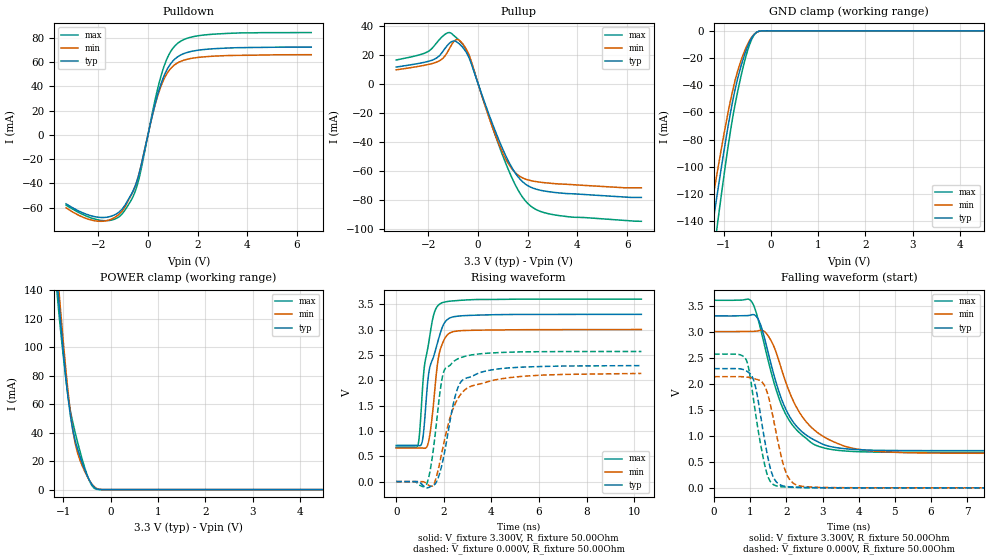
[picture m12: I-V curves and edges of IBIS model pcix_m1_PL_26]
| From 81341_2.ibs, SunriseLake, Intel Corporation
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[Model]   pcix_m1_PL_26
Model_type   I/O
Vinl = 1.155V
Vinh = 1.650V
Vmeas = 1.320V
Vref = 0.000V
Cref = 10.000pF
Rref = 25.000Ohm
|   typ   min   max
C_comp   7.5000pF   6.000pF   9.000pF
[Voltage Range]   3.300V   3.000V   3.600V
[Temperature Range]   60.0   110.0   -5.0
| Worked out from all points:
|   slope of the pulldown table from 0 to 0.495 V, typ, clamps not added: 12.3 ohm
|   slope of the pullup table from 0 to 0.495 V, typ, clamps not added: 20.8 ohm
|   GND clamp passes 1 mA (typ) near -0.30 V on its own axis
|   POWER clamp passes 1 mA (typ) near -0.32 V on its own axis
|   falling waveform, V_fixture 3.300V, R_fixture 50.00Ohm: 20-80 % time 796ps typ, 991ps min, 811ps max; typ from 3.3 V to 0.714 V
|   rising waveform, V_fixture 3.300V, R_fixture 50.00Ohm: 20-80 % time 563ps typ, 338ps min, 429ps max; typ from 0.714 V to 3.3 V
|   rising waveform, V_fixture 0.000V, R_fixture 50.00Ohm: 20-80 % time 596ps typ, 835ps min, 410ps max; typ from 0 V to 2.29 V
|   falling waveform, V_fixture 0.000V, R_fixture 50.00Ohm: 20-80 % time 349ps typ, 405ps min, 362ps max; typ from 2.29 V to 0 V
[Pulldown]
|   Voltage   I(typ)   I(min)   I(max)
-3.3V     -56.89mA   -60.17mA   -57.97mA
-1.9V     -68.16mA   -71.31mA   -70.53mA
-1.35V    -66.03mA   -68.25mA   -69.58mA
-950mV    -58.67mA   -60.17mA   -62.73mA
-600mV    -46.21mA   -46.47mA   -50.78mA
-400mV    -35.07mA   -34.98mA   -39.08mA
200mV     18.27mA    17.98mA    20.69mA
500mV     40.57mA    38.9mA     46.82mA
850mV     56.8mA     53.13mA    66.45mA
1.25V     65.06mA    59.98mA    76.34mA
2.65V     71.02mA    64.89mA    83.04mA
6.575V    72.39mA    66.1mA     84.35mA
[GND Clamp]
|   Voltage   I(typ)   I(min)   I(max)
-3.3V     -632.5mA   -564.4mA   -725.5mA
-1.325V   -165.6mA   -144.4mA   -196mA
-1.3V     -159.5mA   -139mA     -189mA
-1.25V    -147.6mA   -128.4mA   -175.3mA
-1.2V     -135.8mA   -118mA     -161.6mA
-1.125V   -118.5mA   -102.6mA   -141.4mA
-850mV    -59.64mA   -50.8mA    -72.97mA
-650mV    -28.41mA   -23.93mA   -36.31mA
-450mV    -8.219mA   -7.112mA   -10.14mA
-350mV    -2.584mA   -2.413mA   -2.802mA
-250mV    -331.3uA   -398.2uA   -220.5uA
6.575V    0A         0A         0A
[Pullup]
|   Voltage   I(typ)   I(min)   I(max)
-3.3V     11.57mA    9.657mA    16.44mA
-2.15V    14.9mA     12.82mA    21.17mA
-1.65V    18.08mA    15.15mA    28.67mA
-1.1V     28.76mA    26.01mA    35.05mA
-850mV    28.79mA    30.56mA    31.39mA
-500mV    22.31mA    24.52mA    24.17mA
500mV     -24.06mA   -26.25mA   -25.99mA
1V        -45.34mA   -47.85mA   -49.88mA
1.5V      -61.59mA   -61.32mA   -69.74mA
2V        -70.18mA   -66.18mA   -82.46mA
3.2V      -75.08mA   -68.95mA   -90.66mA
6.575V    -78.32mA   -71.68mA   -94.75mA
[POWER Clamp]
|   Voltage   I(typ)   I(min)   I(max)
-3.3V     1.109A     1.089A     1.13A
-1.15V    154.7mA    163.7mA    144.9mA
-1.1V     134.6mA    143.1mA    126.4mA
-1.075V   125mA      133.1mA    118mA
-900mV    64.86mA    68.99mA    65.55mA
-800mV    41.99mA    41.86mA    47.4mA
-750mV    34.63mA    32.54mA    40.32mA
-650mV    23.51mA    20.95mA    27.23mA
-500mV    10.16mA    9.585mA    10.63mA
-400mV    3.792mA    4.116mA    3.102mA
-300mV    590.1uA    959uA      205.5uA
6.575V    0A         0A         0A
[Ramp]
R_load = 50.00Ohm
|   typ   min   max
dV/dt_r   1.373V/595.247ps   1.280V/835.266ps   1.540V/410.341ps
dV/dt_f   1.552V/795.585ps   1.403V/991.104ps   1.752V/810.789ps
[Falling Waveform]
V_fixture = 3.300V
V_fixture_min = 3.000V
V_fixture_max = 3.600V
R_fixture = 50.00Ohm
|   Time   V(typ)   V(min)   V(max)
0s        3.3V       3V         3.6V
1.04ns    3.322V     3.004V     3.573V
1.25ns    3.195V     3.02V      3.152V
1.47ns    2.669V     2.944V     2.518V
1.92ns    1.61V      2.159V     1.502V
2.33ns    1.145V     1.485V     1.079V
2.83ns    898.8mV    1.078V     812.4mV
3.61ns    752.2mV    800.3mV    708.2mV
4.45ns    721.7mV    704.7mV    686.7mV
10.3ns    713.9mV    662mV      679.2mV
[Rising Waveform]
V_fixture = 3.300V
V_fixture_min = 3.000V
V_fixture_max = 3.600V
R_fixture = 50.00Ohm
|   Time   V(typ)   V(min)   V(max)
0s        713.9mV    662mV      679.2mV
910ps     713.7mV    661.6mV    713.2mV
990ps     708.2mV    661.8mV    1.001V
1.12ns    860.2mV    660.7mV    1.935V
1.36ns    2.114V     789.9mV    2.721V
1.58ns    2.477V     1.599V     3.3V
1.72ns    2.714V     2.267V     3.452V
1.85ns    2.926V     2.604V     3.51V
2.62ns    3.266V     2.974V     3.574V
10.3ns    3.3V       3V         3.6V
[Rising Waveform]
V_fixture = 0.000V
V_fixture_min = 0.000V
V_fixture_max = 0.000V
R_fixture = 50.00Ohm
|   Time   V(typ)   V(min)   V(max)
0s        667.5nV    3.876uV    47.12nV
1.27ns    -122.7mV   -38.69mV   -58.92mV
1.43ns    -100.3mV   -86.73mV   228.6mV
1.59ns    -63.65mV   -43.88mV   745.7mV
1.96ns    414.6mV    668.6mV    2.106V
2.25ns    1.164V     1.244V     2.29V
2.56ns    1.812V     1.611V     2.415V
2.85ns    2.024V     1.796V     2.467V
4.2ns     2.217V     2.011V     2.543V
10.3ns    2.289V     2.134V     2.567V
[Falling Waveform]
V_fixture = 0.000V
V_fixture_min = 0.000V
V_fixture_max = 0.000V
R_fixture = 50.00Ohm
|   Time   V(typ)   V(min)   V(max)
0s        2.289V     2.134V     2.567V
890ps     2.246V     2.127V     2.455V
980ps     2.2V       2.118V     2.21V
1.12ns    2.01V      2.094V     1.559V
1.42ns    833.5mV    1.926V     381.3mV
1.57ns    341mV      1.559V     109mV
1.7ns     134.4mV    1.117V     43.19mV
2ns       26.13mV    275.4mV    14.75mV
2.36ns    9.672mV    38.6mV     6.127mV
10.3ns    667.5nV    3.876uV    47.12nV
